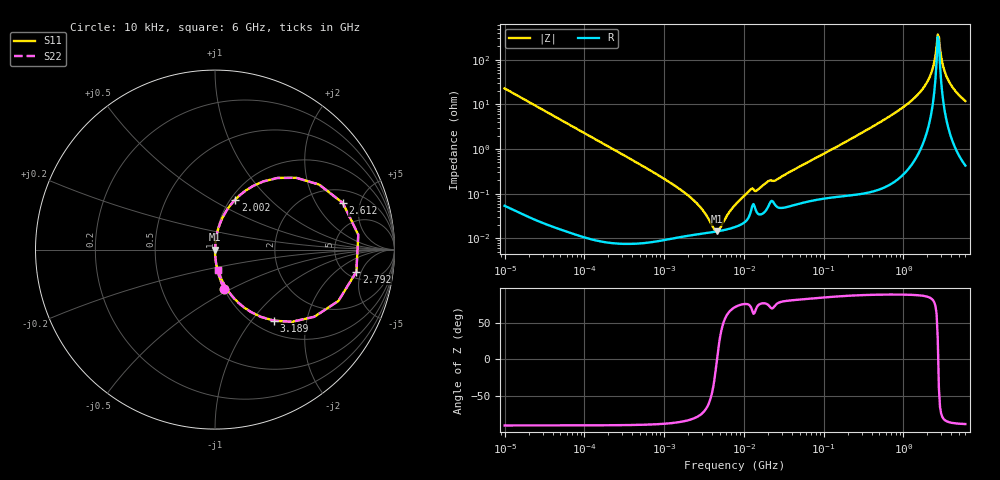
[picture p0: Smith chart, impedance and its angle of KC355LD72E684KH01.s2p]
!Murata Part Number: KC355LD72E684KH01
!These Parameters are Measured in Series Mode Connection
!Data Generated on Jun 19, 2026
!  o--ll--o
!Port1  Port2
!  o------o
!Operation Temp=25[degC], DC Bias Voltage=0[V]
!Freq. Start=10[kHz] Stop=6[GHz] 401[Steps]
# Hz S RI R 50
!Freq.(Hz) S11(Real) S11(Imag) S21(Real) S21(Imag) S12(Real) S12(Imag) S22(Real) S22(Imag)
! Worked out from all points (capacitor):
!   401 points, 10 kHz to 6 GHz, reference 50 ohm
!   read as one part in series: C = 697 nF near 10.69 kHz
!   lowest |Z| = 14.3 mohm at 4.549 MHz (marker M1)
!   series resonance near 4.606 MHz, so ESL is about 1.7 nH
!   S11 on the Smith chart (normalised r, x): 10 kHz: 1.00, -0.46; 2.002 GHz: 1.05, +0.65; 2.612 GHz: 2.84, +3.46; 2.792 GHz: 6.05, -4.08; 3.189 GHz: 1.21, -1.31; 6 GHz: 1.01, -0.24
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10000  0.05 -0.2168  0.95 0.2168  0.95 0.2168  0.05 -0.2168
92862  0.000717 -0.0246  0.9993 0.0246  0.9993 0.0246  0.000717 -0.0246
862344  9.37e-05 -0.00254  0.9999 0.00254  0.9999 0.00254  9.37e-05 -0.00254
2418173  0.000121 -0.000669  0.9999 0.000669  0.9999 0.000669  0.000121 -0.000669
4549352  0.000142 -1.19e-05  0.9999 1.19e-05  0.9999 1.19e-05  0.000142 -1.19e-05
7745967  0.000179 0.000528  0.9998 -0.000528  0.9998 -0.000528  0.000179 0.000528
1.193618e7  0.000348 0.00115  0.9997 -0.00115  0.9997 -0.00115  0.000348 0.00115
1.457263e7  0.000381 0.00112  0.9996 -0.00112  0.9996 -0.00112  0.000381 0.00112
2.032318e7  0.00053 0.00184  0.9995 -0.00184  0.9995 -0.00184  0.00053 0.00184
2.565129e7  0.000522 0.00198  0.9995 -0.00198  0.9995 -0.00198  0.000522 0.00198
7.193098e7  0.000728 0.00565  0.9993 -0.00565  0.9993 -0.00565  0.000728 0.00565
6.67969e8  0.00441 0.0533  0.9956 -0.0533  0.9956 -0.0533  0.00441 0.0533
1.343103e9  0.0223 0.1296  0.9777 -0.1296  0.9777 -0.1296  0.0223 0.1296
2.001953e9  0.1131 0.279  0.8869 -0.279  0.8869 -0.279  0.1131 0.279
2.364181e9  0.3481 0.3991  0.6519 -0.3991  0.6519 -0.3991  0.3481 0.3991
2.612262e9  0.7124 0.2593  0.2876 -0.2593  0.2876 -0.2593  0.7124 0.2593
2.791949e9  0.7876 -0.123  0.2124 0.123  0.2124 0.123  0.7876 -0.123
2.983997e9  0.5531 -0.3744  0.4469 0.3744  0.4469 0.3744  0.5531 -0.3744
3.189254e9  0.3304 -0.3962  0.6696 0.3962  0.6696 0.3962  0.3304 -0.3962
3.523913e9  0.1621 -0.3224  0.8379 0.3224  0.8379 0.3224  0.1621 -0.3224
3.89369e9  0.0911 -0.2541  0.9089 0.2541  0.9089 0.2541  0.0911 -0.2541
6e9  0.018 -0.1161  0.982 0.1161  0.982 0.1161  0.018 -0.1161
